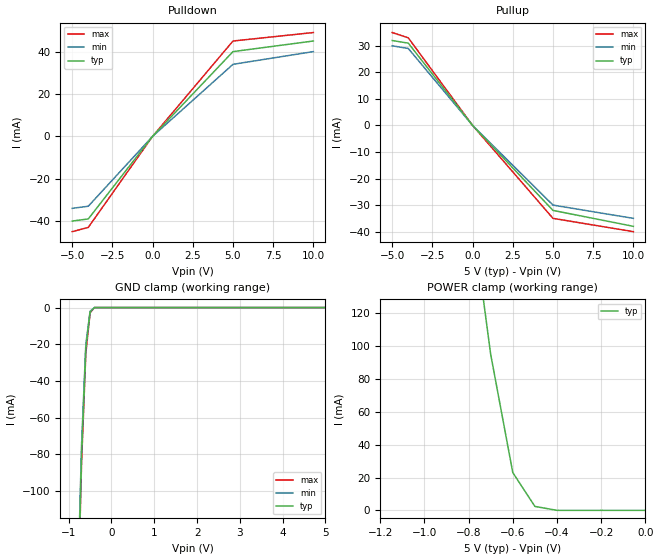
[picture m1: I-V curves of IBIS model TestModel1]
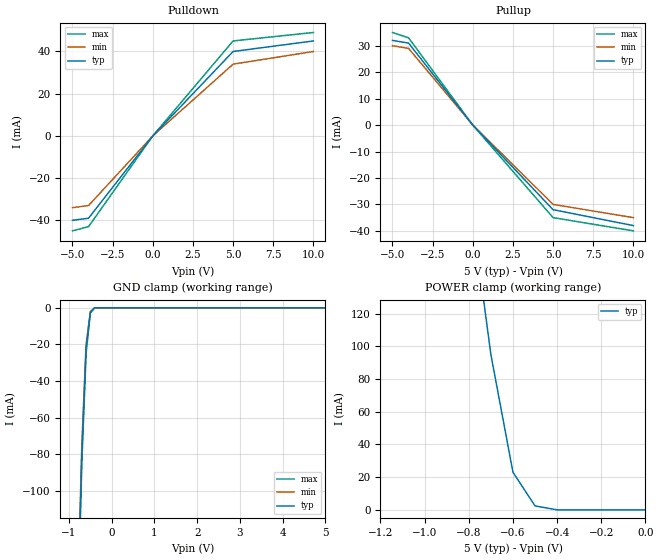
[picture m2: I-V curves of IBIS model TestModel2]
|DESCRIPTION OF BUG:
|Section 6a of the IBIS 3.2 specification states, under the [Submodel]
|keyword usage rules:
|"A .ibs file must contain enough [Submodel] keywords to cover all
|of the model names specified under the [Add Submodel] keyword."
|The current parser will not generate a warning or error if *no*
|[Submodel]s are defined in a file containing one or more [Add Submodel]
|keywords.
|At present, an error *is* generated if one or more correctly-matched
|[Submodel]-[Add Submodel] pairs exists in the file and at least one
|[Submodel] is missing:
|   ERROR - Could not find definition for Submodel xxx of Model yyy
|The same error message should be generated for any file where the
|number of [Submodel] keywords and the number of [Add Submodel]
|keywords do not match.
|This bug also applies to DOS32 IBISCHK3 v3.2.5 under Windows 98SE.
[IBIS Ver]   3.2
[File Name]   bug51.ibs
[File Rev]   0.0
[Date]   05-December-2000
[Source]   File created from specification
[Notes]   Using the IBISCHK3 v3.2.5 parser, the following file
   will generate no errors or warnings.  If one of
   the [Submodel] declarations is un-commented, only
   then will an error regarding the missing [Submodel]
   be generated.
[Disclaimer]
   (C) Copyright 2000 Intel Corp.
   All rights reserved
   This model is for demonstration purposes only,
[Component]   GENERIC_IBIS
[Manufacturer]   Intel Corp.
[Package]
|   typ   min   max
R_pkg   6.0mO   5.0mO   7.0mO
L_pkg   5.0nH   2.0nH   8.0nH
C_pkg   1.0pF   0.5pF   1.5pF
[Pin]   signal_name   model_name   R_pin   L_pin   C_pin
   1   TestSignal1   TestModel1
   2   TestSignal2   TestModel2
| Models and submodels in the file (2): TestModel1 (I/O), TestModel2 (I/O)
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[Model]   TestModel1
Model_type   I/O
Polarity   Non-Inverting
Vinl = 800mV
Vinh = 2.0V
Cref = 10.0pF
Vref = 0.0
Rref = 25
Vmeas = 0.4
C_comp   5.00pF   4.00pF   6.00pF
[Temperature Range]   27.00   100.00   0.00
[Voltage Range]   5.0V   4.75V   5.25V
[Add Submodel]
testsub1   Non-Driving
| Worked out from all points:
|   slope of the pulldown table from 0 to 0.75 V, typ, clamps not added: 125 ohm
|   slope of the pullup table from 0 to 0.75 V, typ, clamps not added: 156 ohm
|   GND clamp passes 1 mA (typ) near -0.44 V on its own axis
|   POWER clamp passes 1 mA (typ) near -0.44 V on its own axis
[Pulldown]
| voltage   I(typ)   I(min)   I(max)
-5V       -40mA      -34mA      -45mA
-4V       -39mA      -33mA      -43mA
0V        0A         0A         0A
5V        40mA       34mA       45mA
10V       45mA       40mA       49mA
[Pullup]
| voltage   I(typ)   I(min)   I(max)
-5V       32mA       30mA       35mA
-4V       31mA       29mA       33mA
0V        0A         0A         0A
5V        -32mA      -30mA      -35mA
10V       -38mA      -35mA      -40mA
[GND Clamp]
| voltage   I(typ)   I(min)   I(max)
-5V       -3.9A      -3.8A      -4A
-700mV    -80mA      -75mA      -85mA
-600mV    -22mA      -20mA      -25mA
-500mV    -2.4mA     -2mA       -2.9mA
-400mV    0A         0A         0A
5V        0A         0A         0A
[Power Clamp]
| voltage   I(typ)   I(min)   I(max)
-5V       4.45A      NA         NA
-700mV    95mA       NA         NA
-600mV    23mA       NA         NA
-500mV    2.4mA      NA         NA
-400mV    0A         NA         NA
0V        0A         NA         NA
[Ramp]
|variable   typ   min   max
dV/dt_r   2.20/1.06n   1.92/1.28n   2.49/650p
dV/dt_f   2.46/1.21n   2.21/1.54n   2.70/770p
R_load = 300ohms
|[Submodel]   testsub1
|Submodel_type  Dynamic_clamp
|[GND Clamp]
| voltage   I(typ)   I(min)   I(max)
|  -5.0000   -40.0m   -34.00m   -45.00m
|  -4.0000   -39.0m   -33.00m   -43.00m
|   0.0000   0.0m   0.00m   0.00m
|   5.0000   40.0m   34.0m   45.00m
|  10.0000   45.0m   40.0m   49.00m
[Model]   TestModel2
Model_type   I/O
Polarity   Non-Inverting
Vinl = 800mV
Vinh = 2.0V
Cref = 10.0pF
Vref = 0.0
Rref = 25
Vmeas = 0.4
C_comp   5.00pF   4.00pF   6.00pF
[Temperature Range]   27.00   100.00   0.00
[Voltage Range]   5.0V   4.75V   5.25V
[Add Submodel]
testsub2   Non-Driving
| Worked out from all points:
|   slope of the pulldown table from 0 to 0.75 V, typ, clamps not added: 125 ohm
|   slope of the pullup table from 0 to 0.75 V, typ, clamps not added: 156 ohm
|   GND clamp passes 1 mA (typ) near -0.44 V on its own axis
|   POWER clamp passes 1 mA (typ) near -0.44 V on its own axis
[Pulldown]
| voltage   I(typ)   I(min)   I(max)
-5V       -40mA      -34mA      -45mA
-4V       -39mA      -33mA      -43mA
0V        0A         0A         0A
5V        40mA       34mA       45mA
10V       45mA       40mA       49mA
[Pullup]
| voltage   I(typ)   I(min)   I(max)
-5V       32mA       30mA       35mA
-4V       31mA       29mA       33mA
0V        0A         0A         0A
5V        -32mA      -30mA      -35mA
10V       -38mA      -35mA      -40mA
[GND Clamp]
| voltage   I(typ)   I(min)   I(max)
-5V       -3.9A      -3.8A      -4A
-700mV    -80mA      -75mA      -85mA
-600mV    -22mA      -20mA      -25mA
-500mV    -2.4mA     -2mA       -2.9mA
-400mV    0A         0A         0A
5V        0A         0A         0A
[Power Clamp]
| voltage   I(typ)   I(min)   I(max)
-5V       4.45A      NA         NA
-700mV    95mA       NA         NA
-600mV    23mA       NA         NA
-500mV    2.4mA      NA         NA
-400mV    0A         NA         NA
0V        0A         NA         NA
[Ramp]
|variable   typ   min   max
dV/dt_r   2.20/1.06n   1.92/1.28n   2.49/650p
dV/dt_f   2.46/1.21n   2.21/1.54n   2.70/770p
R_load = 300ohms
